PROGRAM PRG_MachineDataSave	(*只做参数保存, 没有配方, 需要输入一个文件名(如果有重复, 会把旧文件删除, 会影响其他参数!!), 多个变量要保存成多个文件(名)!!*)
VAR
	fbMachineData		: FB_MachineData;
	eFileType			: E_FileType :=eFileType_BIN;
END_VAR

;
fbMachineData(
	bRunOnCeDevice		:= FALSE,					(* TRUE--CE系统, FALSE--非CE系统*)
	sgFilePath			:= ,						(* 文件路径, 默认是 \Data\Machine\' *)
	sgFileName			:= 'MachineData',			(* 文件名 *)
	eFileType			:= eFileType,
	pMacData			:= ADR(sMacData),			(* 机械参数首地址 *)
	pBakData			:= ADR(_sMacData),			(* 机械参数备份的首地址, 保存上一次的参数值, 用来比较参数是否有变化 *)
	nMacSize			:= SIZEOF(sMacData),		(* 机械参数总字节数 *)
	tAutoSave			:= T#10S,					(* 参数变化后, 延时保存(写文件) *)
	bInitialDone		=> ,
	bDone				=> ,
	bBusy				=> ,
	bError				=> );

END_PROGRAM
